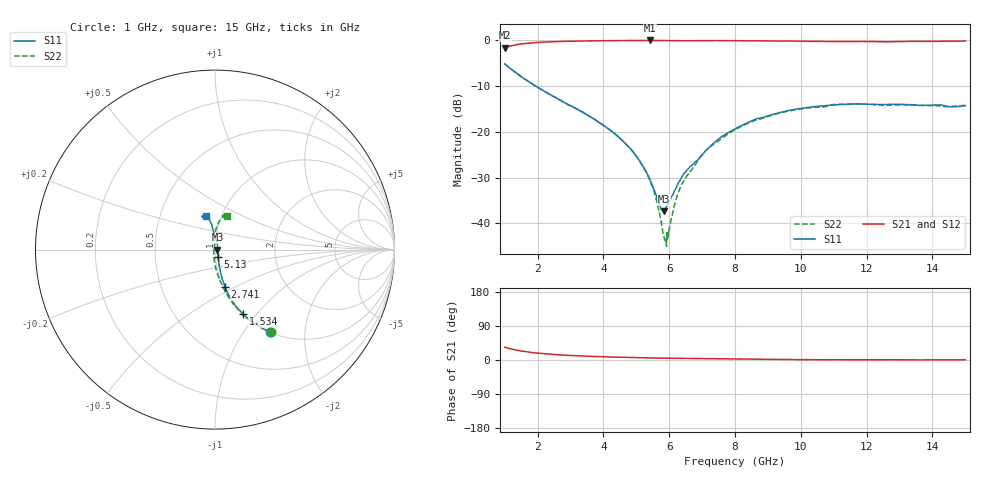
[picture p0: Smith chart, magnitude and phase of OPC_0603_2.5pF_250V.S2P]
! FILE NAME
! DATE 08/14/2012  14:58
! CORRECTED  DATA
# GHz  S  MA  R  50.00
!  FREQ  S11M  S11A  S21M  S21A  S12M  S12A  S22M  S22A
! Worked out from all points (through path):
!   1601 points, 1 GHz to 15 GHz, reference 50 ohm
!   highest |S21| = -0.04 dB at 5.419 GHz (marker M1); lowest = -1.6 dB at 1 GHz (marker M2)
!   group delay of S21, straight-line fit = 3.91 ps
!   lowest |S11| = -37.4 dB at 5.83 GHz (marker M3), VSWR 1.03, Z = 51.4 + j0.0152 ohm
!   |S11| at or under -10 dB: 1.927229 GHz to 1.928831 GHz (1.602 MHz wide, 0.0831 % of centre); 1.941 GHz to end of sweep
!   |S22| runs from -45.0 to -5.1 dB; largest |S21 - S12| = 0.0099
!   S11 on the Smith chart (normalised r, x): 1 GHz: 1.01, -1.33; 1.534 GHz: 1.01, -0.86; 2.741 GHz: 1.02, -0.45; 5.13 GHz: 1.03, -0.09; 15 GHz: 0.84, +0.33
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1  0.553 -56.2  0.8287 33.7  0.8278 33.6  0.5531 -56.0
1.53375  0.3936 -66.4  0.9155 23.3  0.9146 23.2  0.3935 -66.4
2.74125  0.2172 -75.0  0.9715 13.2  0.971 13.1  0.2165 -77.8
3.33625  0.1663 -76.2  0.9821 10.7  0.981 10.6  0.1658 -81.5
4.45625  0.08844 -75.1  0.9925 7.4  0.9918 7.3  0.08757 -89.6
4.85875  0.06324 -71.4  0.994 6.6  0.9931 6.5  0.06279 -93.1
5.13  0.04623 -67.9  0.9952 6.0  0.9939 5.9  0.0461 -96.9
5.41875  0.02997 -58.6  0.996 5.5  0.9945 5.4  0.02907 -104.4
5.55875  0.02246 -48.4  0.9953 5.3  0.9943 5.2  0.02098 -111.0
5.6725  0.01711 -35.1  0.9952 5.0  0.9944 5.0  0.01463 -122.2
5.83  0.01355 0.6  0.9943 4.7  0.9931 4.7  0.007414 -161.7
5.89125  0.01453 15.7  0.9937 4.7  0.9925 4.6  0.006532 168.8
5.935  0.01561 23.9  0.9932 4.6  0.9921 4.5  0.006997 147.7
6.25  0.02635 58.9  0.9909 4.2  0.9896 4.2  0.02049 100.7
6.57375  0.03906 70.8  0.9885 4.0  0.9882 4.0  0.03398 91.9
7.16  0.06488 88.4  0.9915 3.5  0.9902 3.4  0.0643 91.9
8  0.1073 95.2  0.9902 2.5  0.9888 2.5  0.105 88.3
9.155  0.1551 99.3  0.9826 1.6  0.981 1.5  0.1528 82.5
10.33625  0.1872 102.6  0.976 0.8  0.9746 0.7  0.1834 76.9
11.0625  0.1969 104.9  0.969 0.7  0.9678 0.5  0.1991 74.8
12.6725  0.1999 110.3  0.9623 0.6  0.9618 0.4  0.1947 70.8
15  0.1926 105.5  0.9818 0.7  0.9808 0.6  0.1966 70.5
